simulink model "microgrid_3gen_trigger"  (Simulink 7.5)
settings: Solver=ode23tb  StartTime=0.0  StopTime=20  FixedStep=0.001  RelTol=1e-4
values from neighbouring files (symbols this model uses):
  A = [A_ele, -A_ele, 0    [run_microgrid_3gen_trigger.m]
  B = [2*A_ele,-A_ele,A_ele    [run_microgrid_3gen_trigger.m]
  Ereq1 = 1    [run_microgrid_3gen_trigger.m]
  Ereq2 = 1    [run_microgrid_3gen_trigger.m]
  Ereq3 = 1    [run_microgrid_3gen_trigger.m]
  flag_trigger = 0    [run_microgrid_3gen_trigger.m]
  gen_b = [0.1,1.8,0.5]    [run_microgrid_3gen_trigger.m]
  gen_c = [0.1,0.1,0.1]    [run_microgrid_3gen_trigger.m]
  Ki = 750*160    (= 120000)    [run_microgrid_3gen_trigger.m]
  Kilim = 30    [run_microgrid_3gen_trigger.m]
  Kp = 750*0.001    (= 0.75)    [run_microgrid_3gen_trigger.m]
  Kplim = 0    [run_microgrid_3gen_trigger.m]
  Lgen = 0.00188    [run_microgrid_3gen_trigger.m]
  Lline12 = Lline    (= 1.0345071301e-05)    [run_microgrid_3gen_trigger.m]
  Lline23 = Lline    (= 1.0345071301e-05)    [run_microgrid_3gen_trigger.m]
  Lline31 = Lline    (= 1.0345071301e-05)    [run_microgrid_3gen_trigger.m]
  Lload1 = 0.001/w0    (= 2.65258238486e-06)    [run_microgrid_3gen_trigger.m]
  Lload2 = 0.001/w0    (= 2.65258238486e-06)    [run_microgrid_3gen_trigger.m]
  Lload3 = 0.001/w0    (= 2.65258238486e-06)    [run_microgrid_3gen_trigger.m]
  mP = pi    (= 3.14159265359)    [run_microgrid_3gen_trigger.m]
  mQ = 0.05    [run_microgrid_3gen_trigger.m]
  P_lim_d = [-.4,-.4,-.4]    [run_microgrid_3gen_trigger.m]
  P_lim_u = [.4,.4,.4]    [run_microgrid_3gen_trigger.m]
  Pgen_lim_d = [0.0,0.0,0.0]    [run_microgrid_3gen_trigger.m]
  Pgen_lim_u = [1.0,1.0,1.0]    [run_microgrid_3gen_trigger.m]
  Pmax = 1.0    (= 1)    [run_microgrid_3gen_trigger.m]
  Pmin = 0.0    (= 0)    [run_microgrid_3gen_trigger.m]
  Preq1 = 0.4    [run_microgrid_3gen_trigger.m]    (also in odyssian_4a_plot.m = Preq.signals(1).values; Power_Dispatcher.m = 1)
  Preq2 = 0.8    [run_microgrid_3gen_trigger.m]    (also in odyssian_4a_plot.m = Preq.signals(2).values; Power_Dispatcher.m = 1)
  Preq3 = 0.6    [run_microgrid_3gen_trigger.m]    (also in odyssian_4a_plot.m = Preq.signals(3).values; Power_Dispatcher.m = 1)
  Rline12 = Rline    (= 0)    [run_microgrid_3gen_trigger.m]
  Rline23 = Rline    (= 0)    [run_microgrid_3gen_trigger.m]
  Rline31 = Rline    (= 0)    [run_microgrid_3gen_trigger.m]
  Rload1 = 3    [run_microgrid_3gen_trigger.m]
  Rload2 = 4    [run_microgrid_3gen_trigger.m]
  Rload3 = 6    [run_microgrid_3gen_trigger.m]
  Sbase = 15000    [run_microgrid_3gen_trigger.m]
  t_trigger_start = 3    [run_microgrid_3gen_trigger.m]
  tau_Preq = 0.03    [run_microgrid_3gen_trigger.m]
  tauf = 0.03    [run_microgrid_3gen_trigger.m]
  Vbase = 208/sqrt(3)    [run_microgrid_3gen_trigger.m]
  w0 = 2.0*pi*60    (= 376.991118431)    [run_microgrid_3gen_trigger.m]
  w_d_gen = [w_gen,w_gen,w_gen]    [run_microgrid_3gen_trigger.m]
  w_d_link = [w_line;w_line;w_line]    [run_microgrid_3gen_trigger.m]
  w_u_gen = [w_gen,w_gen,w_gen]    [run_microgrid_3gen_trigger.m]
  w_u_link = [w_line;w_line;w_line]    [run_microgrid_3gen_trigger.m]
libraries: powerlib x73, powerlib_extras x3
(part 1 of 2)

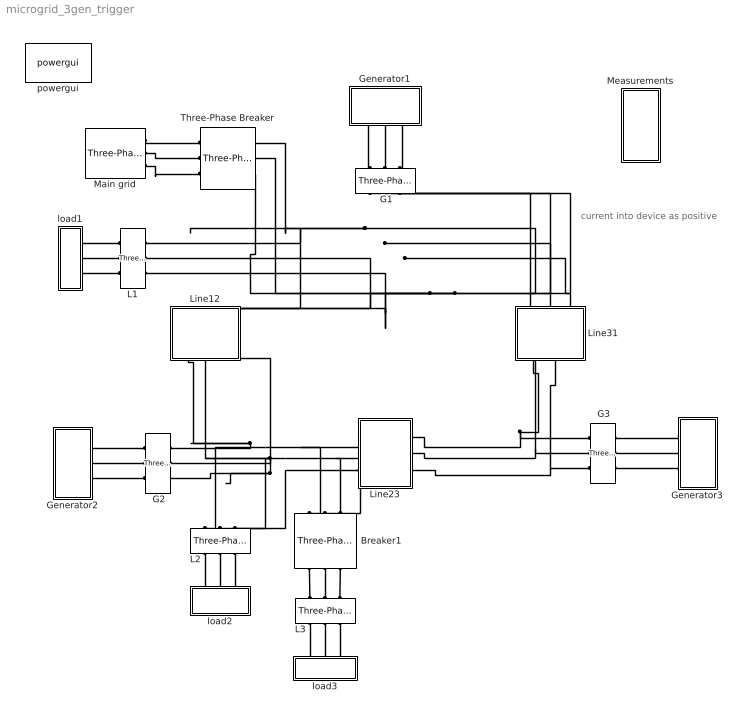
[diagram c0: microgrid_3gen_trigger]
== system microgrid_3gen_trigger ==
  note: current into device as positive
  " G1" : powerlib/Measurements/Three-Phase V-I Measurement  DialogController=POWERSYS.PowerSysDialog  SystemSampleTime=-1  VoltageMeasurement=phase-to-ground  SetLabelV=on  LabelV=v_meas_1  Vpu=off  VpuLL=off  CurrentMeasurement=yes  SetLabelI=on  LabelI=igen_meas_1  Ipu=off  Pbase=100e6  Vbase=500e3  OutputType=Complex  PhasorSimulation=off  PSBequivalent=0
  " G2" : powerlib/Measurements/Three-Phase V-I Measurement  DialogController=POWERSYS.PowerSysDialog  SystemSampleTime=-1  VoltageMeasurement=phase-to-ground  SetLabelV=on  LabelV=v_meas_2  Vpu=off  VpuLL=off  CurrentMeasurement=yes  SetLabelI=on  LabelI=igen_meas_2  Ipu=off  Pbase=100e6  Vbase=500e3  OutputType=Complex  PhasorSimulation=off  PSBequivalent=0
  " G3" : powerlib/Measurements/Three-Phase V-I Measurement  DialogController=POWERSYS.PowerSysDialog  SystemSampleTime=-1  VoltageMeasurement=phase-to-ground  SetLabelV=on  LabelV=v_meas_3  Vpu=off  VpuLL=off  CurrentMeasurement=yes  SetLabelI=on  LabelI=igen_meas_3  Ipu=off  Pbase=100e6  Vbase=500e3  OutputType=Complex  PhasorSimulation=off  PSBequivalent=0
  Breaker1 : powerlib/Elements/Three-Phase Breaker  DialogController=POWERSYS.PowerSysDialog  SystemSampleTime=-1  InitialState=open  SwitchA=on  SwitchB=on  SwitchC=on  SwitchTimes=[10]  External=off  BreakerResistance=0.001  SnubberResistance=1e9  SnubberCapacitance=inf  Measurements=None
  Generator1 : Subsystem
  Generator2 : Subsystem
  Generator3 : Subsystem
  L1 : powerlib/Measurements/Three-Phase V-I Measurement  DialogController=POWERSYS.PowerSysDialog  SystemSampleTime=-1  VoltageMeasurement=phase-to-ground  SetLabelV=on  LabelV=v_meas_load1  Vpu=off  VpuLL=off  CurrentMeasurement=yes  SetLabelI=on  LabelI=iload_meas_1  Ipu=off  Pbase=100e6  Vbase=500e3  OutputType=Complex  PhasorSimulation=off  PSBequivalent=0
  L2 : powerlib/Measurements/Three-Phase V-I Measurement  DialogController=POWERSYS.PowerSysDialog  SystemSampleTime=-1  VoltageMeasurement=phase-to-ground  SetLabelV=on  LabelV=v_meas_load2  Vpu=off  VpuLL=off  CurrentMeasurement=yes  SetLabelI=on  LabelI=iload_meas_2  Ipu=off  Pbase=100e6  Vbase=500e3  OutputType=Complex  PhasorSimulation=off  PSBequivalent=0
  L3 : powerlib/Measurements/Three-Phase V-I Measurement  DialogController=POWERSYS.PowerSysDialog  SystemSampleTime=-1  VoltageMeasurement=phase-to-ground  SetLabelV=on  LabelV=v_meas_load3  Vpu=off  VpuLL=off  CurrentMeasurement=yes  SetLabelI=on  LabelI=iload_meas_3  Ipu=off  Pbase=100e6  Vbase=500e3  OutputType=Complex  PhasorSimulation=off  PSBequivalent=0
  Line12 : Subsystem
  Line23 : Subsystem
  Line31 : Subsystem
  Main grid : powerlib/Electrical Sources/Three-Phase Source  DialogController=POWERSYS.PowerSysDialog  SystemSampleTime=-1  Voltage=208  PhaseAngle=0  Frequency=60  InternalConnection=Yg  SpecifyImpedance=off  Resistance=0.052  Inductance=16.58e-9  ShortCircuitLevel=100e6  BaseVoltage=25e3  XRratio=7
  Measurements : Subsystem
  Three-Phase Breaker : powerlib/Elements/Three-Phase Breaker  DialogController=POWERSYS.PowerSysDialog  SystemSampleTime=-1  InitialState=open  SwitchA=on  SwitchB=on  SwitchC=on  SwitchTimes=[50]  External=off  BreakerResistance=0.001  SnubberResistance=1e9  SnubberCapacitance=inf  Measurements=None
  load1 : Subsystem
  load2 : Subsystem
  load3 : Subsystem
  powergui : powerlib/powergui  Priority=1  SystemSampleTime=-1  SimulationMode=Continuous  SampleTime=50e-6  frequency=60  SPID=off  DisableSnubberDevices=off  DisableRonSwitches=off  DisableVfSwitches=off  SwTol=0  Interpol=off  frequencyindice=0  echomessages=off  HookPort=off  DisplayEquations=off  FunctionMessages=off  EnableUseOfTLC=off  x0status=blocks  RestoreLinks=warning  ResistiveCurrentMeasurement=off  Frange=[0:2:500]  Ylog=off  Xlog=on  ShowGrid=off  save=off  variable=ZData  ZoomFFT=on  StartTime=0.0  cycles=1  DisplayStyle=1  fundamental=60  FreqAxis=off  MaxFrequency=1000  frequencyindicesteady=1  RmsSteady=1  display=off  Ts=0  methode=off
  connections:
  Line23/LConn1 -- Line31/RConn1 -- " G3"/LConn1
  Line23/LConn2 -- Line31/RConn2 -- " G3"/LConn2
  Line23/LConn3 -- Line31/RConn3 -- " G3"/LConn3
  Line23/RConn1 -- " G2"/LConn1 -- Line12/LConn1 -- L2/LConn1 -- Breaker1/LConn1
  Line23/RConn2 -- " G2"/LConn2 -- Line12/LConn2 -- L2/LConn2 -- Breaker1/LConn2
  Line23/RConn3 -- L2/LConn3 -- " G2"/LConn3 -- Line12/LConn3 -- Breaker1/LConn3
  Generator3/RConn3 -- " G3"/RConn3
  Generator3/RConn2 -- " G3"/RConn2
  Generator3/RConn1 -- " G3"/RConn1
  Line31/LConn1 -- " G1"/LConn1 -- L1/LConn1 -- Line12/RConn1 -- Three-Phase Breaker/RConn1
  Line31/LConn2 -- " G1"/LConn2 -- L1/LConn2 -- Line12/RConn2 -- Three-Phase Breaker/RConn2
  Line31/LConn3 -- " G1"/LConn3 -- L1/LConn3 -- Line12/RConn3 -- Three-Phase Breaker/RConn3
  load1/LConn1 -- L1/RConn1
  load1/LConn2 -- L1/RConn2
  load1/LConn3 -- L1/RConn3
  L2/RConn3 -- load2/LConn3
  L2/RConn2 -- load2/LConn2
  L2/RConn1 -- load2/LConn1
  Main grid/RConn1 -- Three-Phase Breaker/LConn1
  Main grid/RConn2 -- Three-Phase Breaker/LConn2
  Main grid/RConn3 -- Three-Phase Breaker/LConn3
  Generator2/RConn2 -- " G2"/RConn2
  Generator2/RConn3 -- " G2"/RConn3
  Generator2/RConn1 -- " G2"/RConn1
  Breaker1/RConn3 -- L3/LConn3
  Breaker1/RConn2 -- L3/LConn2
  Breaker1/RConn1 -- L3/LConn1
  L3/RConn1 -- load3/LConn1
  L3/RConn2 -- load3/LConn2
  L3/RConn3 -- load3/LConn3
  Generator1/RConn2 -- " G1"/RConn2
  Generator1/RConn3 -- " G1"/RConn3
  Generator1/RConn1 -- " G1"/RConn1

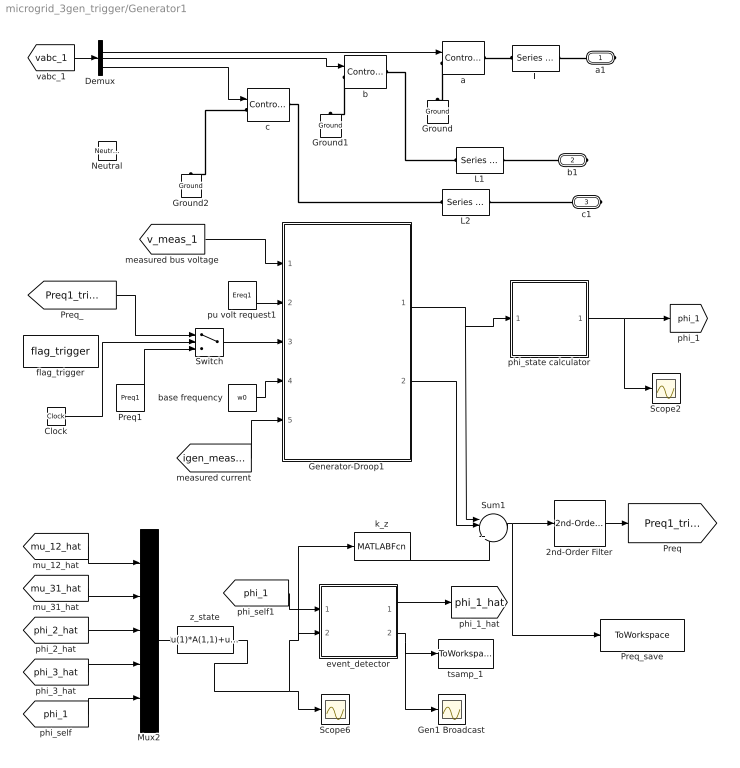
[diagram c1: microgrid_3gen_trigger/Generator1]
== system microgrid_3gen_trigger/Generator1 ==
  2nd-Order Filter : powerlib_extras/Control  Blocks/2nd-Order Filter  DialogController=POWERSYS.PowerSysDialog  SystemSampleTime=-1  FilterType=Lowpass  Fo=20  Zeta=0.707  Initialize=off  Vac_Init=[1 45 60]  Vdc_Init=-0.5  PlotResponse=off  param1=[1 150 1]
  Clock : Clock
  Demux : Demux  Outputs=3
  Gen1 Broadcast : Scope
  Generator-Droop1 : Subsystem
  Ground : powerlib/Elements/Ground  DialogController=POWERSYS.PowerSysDialog  PhysicalDomain=powersysdomain  SubClassName=unknown  LeftPortType=p1  RightPortType=p1  LConnTagsString=a
  Ground1 : powerlib/Elements/Ground  DialogController=POWERSYS.PowerSysDialog  PhysicalDomain=powersysdomain  SubClassName=unknown  LeftPortType=p1  RightPortType=p1  LConnTagsString=a
  Ground2 : powerlib/Elements/Ground  DialogController=POWERSYS.PowerSysDialog  PhysicalDomain=powersysdomain  SubClassName=unknown  LeftPortType=p1  RightPortType=p1  LConnTagsString=a
  L : powerlib/Elements/Series RLC Branch  DialogController=POWERSYS.PowerSysDialog  PhysicalDomain=powersysdomain  SubClassName=unknown  LeftPortType=p1  RightPortType=p1  LConnTagsString=__new0  RConnTagsString=__new0  BranchType=L  Resistance=1  Inductance=Lgen  SetiL0=off  InitialCurrent=0  Capacitance=1e-6  Setx0=off  InitialVoltage=0  Measurements=None
  L1 : powerlib/Elements/Series RLC Branch  DialogController=POWERSYS.PowerSysDialog  PhysicalDomain=powersysdomain  SubClassName=unknown  LeftPortType=p1  RightPortType=p1  LConnTagsString=__new0  RConnTagsString=__new0  BranchType=L  Resistance=1  Inductance=Lgen  SetiL0=off  InitialCurrent=0  Capacitance=1e-6  Setx0=off  InitialVoltage=0  Measurements=None
  L2 : powerlib/Elements/Series RLC Branch  DialogController=POWERSYS.PowerSysDialog  PhysicalDomain=powersysdomain  SubClassName=unknown  LeftPortType=p1  RightPortType=p1  LConnTagsString=__new0  RConnTagsString=__new0  BranchType=L  Resistance=1  Inductance=Lgen  SetiL0=off  InitialCurrent=0  Capacitance=1e-6  Setx0=off  InitialVoltage=0  Measurements=None
  Mux2 : Mux  Inputs=5
  Neutral : powerlib/Elements/Neutral  DialogController=POWERSYS.PowerSysDialog  PhysicalDomain=powersysdomain  SubClassName=unknown  LeftPortType=p1  RightPortType=p1  LConnTagsString=a  NodeNumber=10
  Preq1 : Constant  Value=Preq1  OutDataType=sfix(16)  OutScaling=2^0
  Preq_save : ToWorkspace  VariableName=Preq1_trigger  SampleTime=-1  SaveFormat=Array
  Scope2 : Scope
  Scope6 : Scope
  Sum1 : Sum  Inputs=|++++  OutDataType=sfix(16)  OutScaling=2^0
  Switch : Switch  Criteria=u2 > Threshold  Threshold=t_trigger_start  OutDataType=fixdt(1, 16)  OutScaling=2^0
  a : powerlib/Electrical Sources/Controlled Voltage Source  DialogController=POWERSYS.PowerSysDialog  SystemSampleTime=-1  Initialize=on  Source_Type=AC  Amplitude=0  Phase=0  Frequency=0  Measurements=None
  b : powerlib/Electrical Sources/Controlled Voltage Source  DialogController=POWERSYS.PowerSysDialog  SystemSampleTime=-1  Initialize=on  Source_Type=AC  Amplitude=0  Phase=0  Frequency=0  Measurements=None
  base frequency : Constant  Value=w0  OutDataType=sfix(16)  OutScaling=2^0
  c : powerlib/Electrical Sources/Controlled Voltage Source  DialogController=POWERSYS.PowerSysDialog  SystemSampleTime=-1  Initialize=on  Source_Type=AC  Amplitude=0  Phase=0  Frequency=0  Measurements=None
  event_detector : Subsystem
  flag_trigger : Constant  Value=flag_trigger  OutDataType=sfix(16)  OutScaling=2^0
  k_z : MATLABFcn  MATLABFcn=k_z
  phi_state calculator : Subsystem
  pu volt request1 : Constant  Value=Ereq1  OutDataType=sfix(16)  OutScaling=2^0
  tsamp_1 : ToWorkspace  VariableName=tsamp_1  SampleTime=-1  SaveFormat=Array
  z_state : Fcn  Expr=u(1)*A(1,1)+u(2)*A(3,1)+u(3)*B(2,1)+u(4)*B(3,1)+u(5)*B(1,1)
  a1 : PMIOPort  Port=1  Side=Right
  b1 : PMIOPort  Port=2  Side=Right
  c1 : PMIOPort  Port=3  Side=Right
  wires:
  Demux/1 -> a/1
  Demux/2 -> b/1
  Demux/3 -> c/1
  [vabc_1] -> Demux/1
  pu volt request1/1 -> Generator-Droop1/2(E_req)
  base frequency/1 -> Generator-Droop1/4(w0)
  [v_meas_1] -> Generator-Droop1/1(v_bus_meas)
  [igen_meas_1] -> Generator-Droop1/5(i_meas)
  Generator-Droop1/1(Pmeas) -> Sum1/1, phi_state calculator/1(P_meas)
  [phi_1] -> event_detector/1(phi)
  event_detector/1(phi_hat) -> [phi_1_hat]
  event_detector/2(tsamp) -> tsamp_1/1, Gen1 Broadcast/1
  Sum1/1 -> Preq_save/1, 2nd-Order Filter/1
  Switch/1 -> Generator-Droop1/3(P_req)
  Preq1/1 -> Switch/3
  [Preq1_trigger] -> Switch/1
  Clock/1 -> Switch/2
  phi_state calculator/1(phi) -> [phi_1], Scope2/1
  z_state/1 -> Scope6/1, event_detector/2(z), k_z/1
  k_z/1 -> Sum1/4
  ? -> Sum1/3
  Generator-Droop1/2(Pmm) -> Sum1/2
  2nd-Order Filter/1 -> [Preq1_trigger]
  [mu_12_hat] -> Mux2/1
  [mu_31_hat] -> Mux2/2
  [phi_2_hat] -> Mux2/3
  [phi_3_hat] -> Mux2/4
  [phi_1] -> Mux2/5
  Mux2/1 -> z_state/1
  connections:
  L/RConn1 -- a1/RConn1
  L/LConn1 -- a/RConn1
  L1/RConn1 -- b1/RConn1
  b/RConn1 -- L1/LConn1
  L2/RConn1 -- c1/RConn1
  c/RConn1 -- L2/LConn1
  c/LConn1 -- Ground2/LConn1
  b/LConn1 -- Ground1/LConn1
  a/LConn1 -- Ground/LConn1

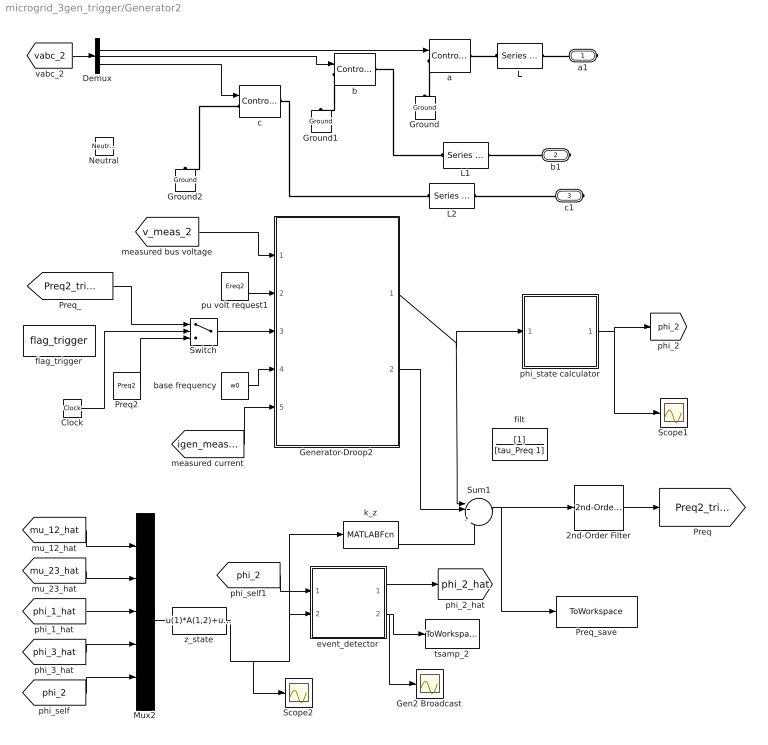
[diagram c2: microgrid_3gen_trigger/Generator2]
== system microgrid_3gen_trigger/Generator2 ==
  2nd-Order Filter : powerlib_extras/Control  Blocks/2nd-Order Filter  DialogController=POWERSYS.PowerSysDialog  SystemSampleTime=-1  FilterType=Lowpass  Fo=20  Zeta=0.707  Initialize=off  Vac_Init=[1 45 60]  Vdc_Init=-0.5  PlotResponse=off  param1=[1 150 1]
  Clock : Clock
  Demux : Demux  Outputs=3
  Gen2 Broadcast : Scope
  Generator-Droop2 : Subsystem
  Ground : powerlib/Elements/Ground  DialogController=POWERSYS.PowerSysDialog  PhysicalDomain=powersysdomain  SubClassName=unknown  LeftPortType=p1  RightPortType=p1  LConnTagsString=a
  Ground1 : powerlib/Elements/Ground  DialogController=POWERSYS.PowerSysDialog  PhysicalDomain=powersysdomain  SubClassName=unknown  LeftPortType=p1  RightPortType=p1  LConnTagsString=a
  Ground2 : powerlib/Elements/Ground  DialogController=POWERSYS.PowerSysDialog  PhysicalDomain=powersysdomain  SubClassName=unknown  LeftPortType=p1  RightPortType=p1  LConnTagsString=a
  L : powerlib/Elements/Series RLC Branch  DialogController=POWERSYS.PowerSysDialog  PhysicalDomain=powersysdomain  SubClassName=unknown  LeftPortType=p1  RightPortType=p1  LConnTagsString=__new0  RConnTagsString=__new0  BranchType=L  Resistance=1  Inductance=Lgen  SetiL0=off  InitialCurrent=0  Capacitance=1e-6  Setx0=off  InitialVoltage=0  Measurements=None
  L1 : powerlib/Elements/Series RLC Branch  DialogController=POWERSYS.PowerSysDialog  PhysicalDomain=powersysdomain  SubClassName=unknown  LeftPortType=p1  RightPortType=p1  LConnTagsString=__new0  RConnTagsString=__new0  BranchType=L  Resistance=1  Inductance=Lgen  SetiL0=off  InitialCurrent=0  Capacitance=1e-6  Setx0=off  InitialVoltage=0  Measurements=None
  L2 : powerlib/Elements/Series RLC Branch  DialogController=POWERSYS.PowerSysDialog  PhysicalDomain=powersysdomain  SubClassName=unknown  LeftPortType=p1  RightPortType=p1  LConnTagsString=__new0  RConnTagsString=__new0  BranchType=L  Resistance=1  Inductance=Lgen  SetiL0=off  InitialCurrent=0  Capacitance=1e-6  Setx0=off  InitialVoltage=0  Measurements=None
  Mux2 : Mux  Inputs=5
  Neutral : powerlib/Elements/Neutral  DialogController=POWERSYS.PowerSysDialog  PhysicalDomain=powersysdomain  SubClassName=unknown  LeftPortType=p1  RightPortType=p1  LConnTagsString=a  NodeNumber=10
  Preq2 : Constant  Value=Preq2  OutDataType=sfix(16)  OutScaling=2^0
  Preq_save : ToWorkspace  VariableName=Preq2_trigger  SampleTime=-1  SaveFormat=Array
  Scope1 : Scope
  Scope2 : Scope
  Sum1 : Sum  Inputs=|++++  OutDataType=sfix(16)  OutScaling=2^0
  Switch : Switch  Criteria=u2 > Threshold  Threshold=t_trigger_start  OutDataType=fixdt(1, 16)  OutScaling=2^0
  a : powerlib/Electrical Sources/Controlled Voltage Source  DialogController=POWERSYS.PowerSysDialog  SystemSampleTime=-1  Initialize=on  Source_Type=AC  Amplitude=0  Phase=0  Frequency=0  Measurements=None
  b : powerlib/Electrical Sources/Controlled Voltage Source  DialogController=POWERSYS.PowerSysDialog  SystemSampleTime=-1  Initialize=on  Source_Type=AC  Amplitude=0  Phase=0  Frequency=0  Measurements=None
  base frequency : Constant  Value=w0  OutDataType=sfix(16)  OutScaling=2^0
  c : powerlib/Electrical Sources/Controlled Voltage Source  DialogController=POWERSYS.PowerSysDialog  SystemSampleTime=-1  Initialize=on  Source_Type=AC  Amplitude=0  Phase=0  Frequency=0  Measurements=None
  event_detector : Subsystem
  filt : TransferFcn  Denominator=[tau_Preq 1]
  flag_trigger : Constant  Value=flag_trigger  OutDataType=sfix(16)  OutScaling=2^0
  k_z : MATLABFcn  MATLABFcn=k_z
  phi_state calculator : Subsystem
  pu volt request1 : Constant  Value=Ereq2  OutDataType=sfix(16)  OutScaling=2^0
  tsamp_2 : ToWorkspace  VariableName=tsamp_2  SampleTime=-1  SaveFormat=Array
  z_state : Fcn  Expr=u(1)*A(1,2)+u(2)*A(2,2)+u(3)*B(1,2)+u(4)*B(3,2)+u(5)*B(2,2)
  a1 : PMIOPort  Port=1  Side=Right
  b1 : PMIOPort  Port=2  Side=Right
  c1 : PMIOPort  Port=3  Side=Right
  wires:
  Demux/1 -> a/1
  Demux/2 -> b/1
  Demux/3 -> c/1
  [vabc_2] -> Demux/1
  pu volt request1/1 -> Generator-Droop2/2(E_req)
  base frequency/1 -> Generator-Droop2/4(w0)
  [v_meas_2] -> Generator-Droop2/1(v_bus_meas)
  [igen_meas_2] -> Generator-Droop2/5(i_meas)
  Generator-Droop2/1(Pmeas) -> Sum1/1, phi_state calculator/1(P_meas)
  [phi_2] -> event_detector/1(phi)
  event_detector/1(phi_hat) -> [phi_2_hat]
  event_detector/2(tsamp) -> tsamp_2/1, Gen2 Broadcast/1
  Sum1/1 -> Preq_save/1, 2nd-Order Filter/1
  Switch/1 -> Generator-Droop2/3(P_req)
  Preq2/1 -> Switch/3
  [Preq2_trigger] -> Switch/1
  Clock/1 -> Switch/2
  phi_state calculator/1(phi) -> [phi_2], Scope1/1
  z_state/1 -> event_detector/2(z), k_z/1, Scope2/1
  k_z/1 -> Sum1/4
  ? -> Sum1/3
  Generator-Droop2/2(Pmm) -> Sum1/2
  2nd-Order Filter/1 -> [Preq2_trigger]
  [mu_12_hat] -> Mux2/1
  [mu_23_hat] -> Mux2/2
  [phi_1_hat] -> Mux2/3
  [phi_3_hat] -> Mux2/4
  [phi_2] -> Mux2/5
  Mux2/1 -> z_state/1
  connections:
  L/RConn1 -- a1/RConn1
  L/LConn1 -- a/RConn1
  L1/RConn1 -- b1/RConn1
  b/RConn1 -- L1/LConn1
  L2/RConn1 -- c1/RConn1
  c/RConn1 -- L2/LConn1
  c/LConn1 -- Ground2/LConn1
  b/LConn1 -- Ground1/LConn1
  a/LConn1 -- Ground/LConn1

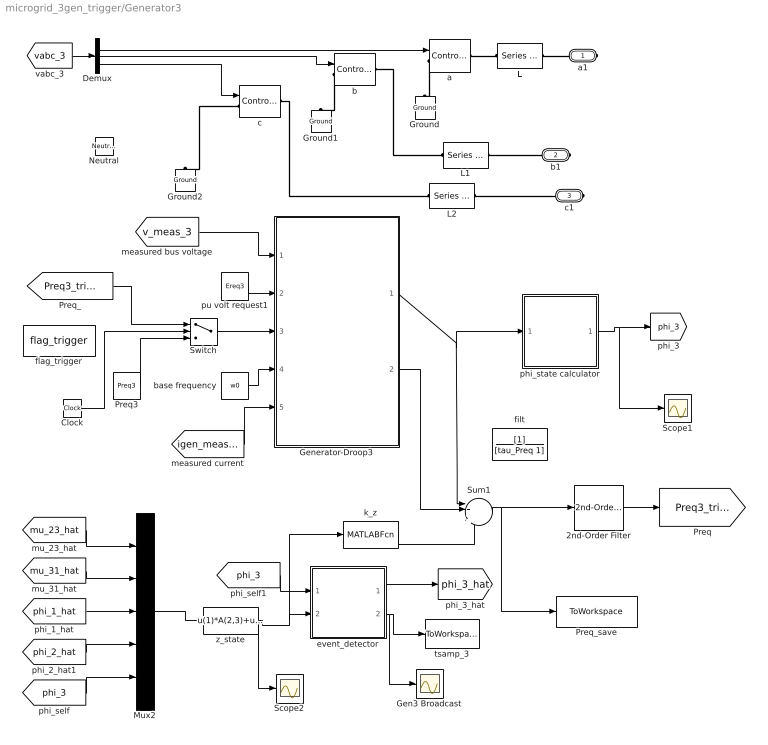
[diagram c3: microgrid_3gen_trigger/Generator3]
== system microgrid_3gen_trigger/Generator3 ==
  2nd-Order Filter : powerlib_extras/Control  Blocks/2nd-Order Filter  DialogController=POWERSYS.PowerSysDialog  SystemSampleTime=-1  FilterType=Lowpass  Fo=20  Zeta=0.707  Initialize=off  Vac_Init=[1 45 60]  Vdc_Init=-0.5  PlotResponse=off  param1=[1 150 1]
  Clock : Clock
  Demux : Demux  Outputs=3
  Gen3 Broadcast : Scope
  Generator-Droop3 : Subsystem
  Ground : powerlib/Elements/Ground  DialogController=POWERSYS.PowerSysDialog  PhysicalDomain=powersysdomain  SubClassName=unknown  LeftPortType=p1  RightPortType=p1  LConnTagsString=a
  Ground1 : powerlib/Elements/Ground  DialogController=POWERSYS.PowerSysDialog  PhysicalDomain=powersysdomain  SubClassName=unknown  LeftPortType=p1  RightPortType=p1  LConnTagsString=a
  Ground2 : powerlib/Elements/Ground  DialogController=POWERSYS.PowerSysDialog  PhysicalDomain=powersysdomain  SubClassName=unknown  LeftPortType=p1  RightPortType=p1  LConnTagsString=a
  L : powerlib/Elements/Series RLC Branch  DialogController=POWERSYS.PowerSysDialog  PhysicalDomain=powersysdomain  SubClassName=unknown  LeftPortType=p1  RightPortType=p1  LConnTagsString=__new0  RConnTagsString=__new0  BranchType=L  Resistance=1  Inductance=Lgen  SetiL0=off  InitialCurrent=0  Capacitance=1e-6  Setx0=off  InitialVoltage=0  Measurements=None
  L1 : powerlib/Elements/Series RLC Branch  DialogController=POWERSYS.PowerSysDialog  PhysicalDomain=powersysdomain  SubClassName=unknown  LeftPortType=p1  RightPortType=p1  LConnTagsString=__new0  RConnTagsString=__new0  BranchType=L  Resistance=1  Inductance=Lgen  SetiL0=off  InitialCurrent=0  Capacitance=1e-6  Setx0=off  InitialVoltage=0  Measurements=None
  L2 : powerlib/Elements/Series RLC Branch  DialogController=POWERSYS.PowerSysDialog  PhysicalDomain=powersysdomain  SubClassName=unknown  LeftPortType=p1  RightPortType=p1  LConnTagsString=__new0  RConnTagsString=__new0  BranchType=L  Resistance=1  Inductance=Lgen  SetiL0=off  InitialCurrent=0  Capacitance=1e-6  Setx0=off  InitialVoltage=0  Measurements=None
  Mux2 : Mux  Inputs=5
  Neutral : powerlib/Elements/Neutral  DialogController=POWERSYS.PowerSysDialog  PhysicalDomain=powersysdomain  SubClassName=unknown  LeftPortType=p1  RightPortType=p1  LConnTagsString=a  NodeNumber=10
  Preq3 : Constant  Value=Preq3  OutDataType=sfix(16)  OutScaling=2^0
  Preq_save : ToWorkspace  VariableName=Preq3_trigger  SampleTime=-1  SaveFormat=Array
  Scope1 : Scope
  Scope2 : Scope
  Sum1 : Sum  Inputs=|++++  OutDataType=sfix(16)  OutScaling=2^0
  Switch : Switch  Criteria=u2 > Threshold  Threshold=t_trigger_start  OutDataType=fixdt(1, 16)  OutScaling=2^0
  a : powerlib/Electrical Sources/Controlled Voltage Source  DialogController=POWERSYS.PowerSysDialog  SystemSampleTime=-1  Initialize=on  Source_Type=AC  Amplitude=0  Phase=0  Frequency=0  Measurements=None
  b : powerlib/Electrical Sources/Controlled Voltage Source  DialogController=POWERSYS.PowerSysDialog  SystemSampleTime=-1  Initialize=on  Source_Type=AC  Amplitude=0  Phase=0  Frequency=0  Measurements=None
  base frequency : Constant  Value=w0  OutDataType=sfix(16)  OutScaling=2^0
  c : powerlib/Electrical Sources/Controlled Voltage Source  DialogController=POWERSYS.PowerSysDialog  SystemSampleTime=-1  Initialize=on  Source_Type=AC  Amplitude=0  Phase=0  Frequency=0  Measurements=None
  event_detector : Subsystem
  filt : TransferFcn  Denominator=[tau_Preq 1]
  flag_trigger : Constant  Value=flag_trigger  OutDataType=sfix(16)  OutScaling=2^0
  k_z : MATLABFcn  MATLABFcn=k_z
  phi_state calculator : Subsystem
  pu volt request1 : Constant  Value=Ereq3  OutDataType=sfix(16)  OutScaling=2^0
  tsamp_3 : ToWorkspace  VariableName=tsamp_3  SampleTime=-1  SaveFormat=Array
  z_state : Fcn  Expr=u(1)*A(2,3)+u(2)*A(3,3)+u(3)*B(1,3)+u(4)*B(2,3)+u(5)*B(3,3)
  a1 : PMIOPort  Port=1  Side=Right
  b1 : PMIOPort  Port=2  Side=Right
  c1 : PMIOPort  Port=3  Side=Right
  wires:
  Demux/1 -> a/1
  Demux/2 -> b/1
  Demux/3 -> c/1
  [vabc_3] -> Demux/1
  pu volt request1/1 -> Generator-Droop3/2(E_req)
  base frequency/1 -> Generator-Droop3/4(w0)
  [v_meas_3] -> Generator-Droop3/1(v_bus_meas)
  [igen_meas_3] -> Generator-Droop3/5(i_meas)
  Generator-Droop3/1(Pmeas) -> Sum1/1, phi_state calculator/1(P_meas)
  [phi_3] -> event_detector/1(phi)
  event_detector/1(phi_hat) -> [phi_3_hat]
  event_detector/2(tsamp) -> tsamp_3/1, Gen3 Broadcast/1
  Sum1/1 -> Preq_save/1, 2nd-Order Filter/1
  Switch/1 -> Generator-Droop3/3(P_req)
  Preq3/1 -> Switch/3
  [Preq3_trigger] -> Switch/1
  Clock/1 -> Switch/2
  phi_state calculator/1(phi) -> [phi_3], Scope1/1
  z_state/1 -> event_detector/2(z), k_z/1, Scope2/1
  k_z/1 -> Sum1/4
  ? -> Sum1/3
  Generator-Droop3/2(Pmm) -> Sum1/2
  2nd-Order Filter/1 -> [Preq3_trigger]
  [mu_23_hat] -> Mux2/1
  [mu_31_hat] -> Mux2/2
  [phi_1_hat] -> Mux2/3
  [phi_2_hat] -> Mux2/4
  [phi_3] -> Mux2/5
  Mux2/1 -> z_state/1
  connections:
  L/RConn1 -- a1/RConn1
  L/LConn1 -- a/RConn1
  L1/RConn1 -- b1/RConn1
  b/RConn1 -- L1/LConn1
  L2/RConn1 -- c1/RConn1
  c/RConn1 -- L2/LConn1
  c/LConn1 -- Ground2/LConn1
  b/LConn1 -- Ground1/LConn1
  a/LConn1 -- Ground/LConn1

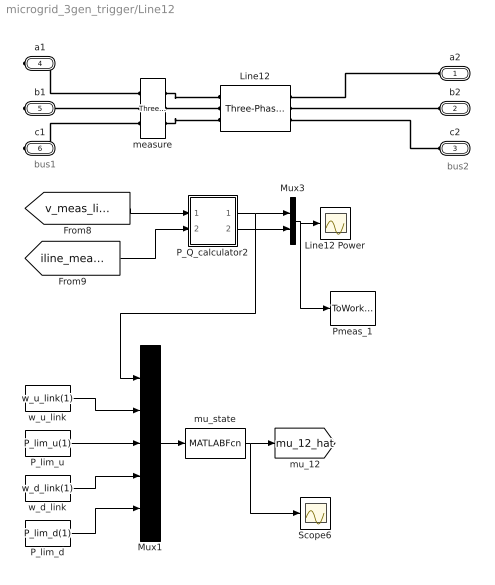
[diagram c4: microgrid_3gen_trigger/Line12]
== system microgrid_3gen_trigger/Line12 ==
  note: bus1
  note: bus2
  Line12 : powerlib/Elements/Three-Phase Series RLC Branch  DialogController=POWERSYS.PowerSysDialog  PhysicalDomain=powersysdomain  SubClassName=unknown  LeftPortType=p1  RightPortType=p1  LConnTagsString=A|B|C  RConnTagsString=A|B|C  BranchType=RL  Resistance=Rline12  Inductance=Lline12  Capacitance=1e-6  Measurements=None
  Line12 Power : Scope
  Mux1 : Mux  Inputs=5
  Mux3 : Mux  Inputs=2
  P_Q_calculator2 : Subsystem
  P_lim_d : Constant  Value=P_lim_d(1)  OutDataType=sfix(16)  OutScaling=2^0
  P_lim_u : Constant  Value=P_lim_u(1)  OutDataType=sfix(16)  OutScaling=2^0
  Pmeas_1 : ToWorkspace  VariableName=PQline_12  SampleTime=-1  SaveFormat=Array
  Scope6 : Scope
  measure : powerlib/Measurements/Three-Phase V-I Measurement  DialogController=POWERSYS.PowerSysDialog  SystemSampleTime=-1  VoltageMeasurement=phase-to-ground  SetLabelV=on  LabelV=v_meas_line12  Vpu=off  VpuLL=off  CurrentMeasurement=yes  SetLabelI=on  LabelI=iline_meas_12  Ipu=off  Pbase=100e6  Vbase=500e3  OutputType=Complex  PhasorSimulation=off  PSBequivalent=0
  mu_state : MATLABFcn  MATLABFcn=mu_state
  w_d_link : Constant  Value=w_d_link(1)  OutDataType=sfix(16)  OutScaling=2^0
  w_u_link : Constant  Value=w_u_link(1)  OutDataType=sfix(16)  OutScaling=2^0
  a2 : PMIOPort  Port=1  Side=Left
  b2 : PMIOPort  Port=2  Side=Left
  c2 : PMIOPort  Port=3  Side=Left
  a1 : PMIOPort  Port=4  Side=Right
  b1 : PMIOPort  Port=5  Side=Right
  c1 : PMIOPort  Port=6  Side=Right
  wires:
  [v_meas_line12] -> P_Q_calculator2/1(v)
  [iline_meas_12] -> P_Q_calculator2/2(i)
  Mux3/1 -> Line12 Power/1, Pmeas_1/1
  P_Q_calculator2/1(P) -> Mux3/1, Mux1/1
  P_Q_calculator2/2(Q) -> Mux3/2
  Mux1/1 -> mu_state/1
  w_u_link/1 -> Mux1/2
  P_lim_u/1 -> Mux1/3
  w_d_link/1 -> Mux1/4
  P_lim_d/1 -> Mux1/5
  mu_state/1 -> [mu_12_hat], Scope6/1
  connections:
  Line12/LConn1 -- a2/RConn1
  Line12/LConn2 -- b2/RConn1
  Line12/LConn3 -- c2/RConn1
  measure/RConn1 -- Line12/RConn1
  measure/RConn2 -- Line12/RConn2
  measure/RConn3 -- Line12/RConn3
  a1/RConn1 -- measure/LConn1
  b1/RConn1 -- measure/LConn2
  c1/RConn1 -- measure/LConn3

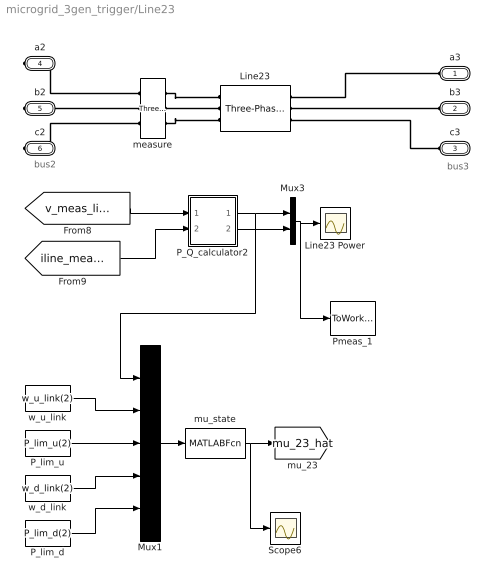
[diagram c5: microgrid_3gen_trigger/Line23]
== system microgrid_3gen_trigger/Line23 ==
  note: bus2
  note: bus3
  Line23 : powerlib/Elements/Three-Phase Series RLC Branch  DialogController=POWERSYS.PowerSysDialog  PhysicalDomain=powersysdomain  SubClassName=unknown  LeftPortType=p1  RightPortType=p1  LConnTagsString=A|B|C  RConnTagsString=A|B|C  BranchType=RL  Resistance=Rline23  Inductance=Lline23  Capacitance=1e-6  Measurements=None
  Line23 Power : Scope
  Mux1 : Mux  Inputs=5
  Mux3 : Mux  Inputs=2
  P_Q_calculator2 : Subsystem
  P_lim_d : Constant  Value=P_lim_d(2)  OutDataType=sfix(16)  OutScaling=2^0
  P_lim_u : Constant  Value=P_lim_u(2)  OutDataType=sfix(16)  OutScaling=2^0
  Pmeas_1 : ToWorkspace  VariableName=PQline_23  SampleTime=-1  SaveFormat=Array
  Scope6 : Scope
  measure : powerlib/Measurements/Three-Phase V-I Measurement  DialogController=POWERSYS.PowerSysDialog  SystemSampleTime=-1  VoltageMeasurement=phase-to-ground  SetLabelV=on  LabelV=v_meas_line23  Vpu=off  VpuLL=off  CurrentMeasurement=yes  SetLabelI=on  LabelI=iline_meas_23  Ipu=off  Pbase=100e6  Vbase=500e3  OutputType=Complex  PhasorSimulation=off  PSBequivalent=0
  mu_state : MATLABFcn  MATLABFcn=mu_state
  w_d_link : Constant  Value=w_d_link(2)  OutDataType=sfix(16)  OutScaling=2^0
  w_u_link : Constant  Value=w_u_link(2)  OutDataType=sfix(16)  OutScaling=2^0
  a3 : PMIOPort  Port=1  Side=Left
  b3 : PMIOPort  Port=2  Side=Left
  c3 : PMIOPort  Port=3  Side=Left
  a2 : PMIOPort  Port=4  Side=Right
  b2 : PMIOPort  Port=5  Side=Right
  c2 : PMIOPort  Port=6  Side=Right
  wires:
  [v_meas_line23] -> P_Q_calculator2/1(v)
  [iline_meas_23] -> P_Q_calculator2/2(i)
  Mux3/1 -> Line23 Power/1, Pmeas_1/1
  P_Q_calculator2/1(P) -> Mux3/1, Mux1/1
  P_Q_calculator2/2(Q) -> Mux3/2
  Mux1/1 -> mu_state/1
  w_u_link/1 -> Mux1/2
  P_lim_u/1 -> Mux1/3
  w_d_link/1 -> Mux1/4
  P_lim_d/1 -> Mux1/5
  mu_state/1 -> [mu_23_hat], Scope6/1
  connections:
  Line23/LConn1 -- a3/RConn1
  Line23/LConn2 -- b3/RConn1
  Line23/LConn3 -- c3/RConn1
  measure/RConn1 -- Line23/RConn1
  measure/RConn2 -- Line23/RConn2
  measure/RConn3 -- Line23/RConn3
  a2/RConn1 -- measure/LConn1
  b2/RConn1 -- measure/LConn2
  c2/RConn1 -- measure/LConn3

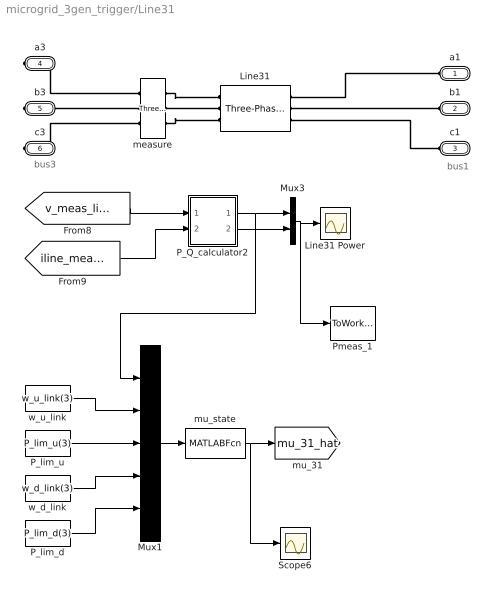
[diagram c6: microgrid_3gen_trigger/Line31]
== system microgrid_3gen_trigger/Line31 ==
  note: bus3
  note: bus1
  Line31 : powerlib/Elements/Three-Phase Series RLC Branch  DialogController=POWERSYS.PowerSysDialog  PhysicalDomain=powersysdomain  SubClassName=unknown  LeftPortType=p1  RightPortType=p1  LConnTagsString=A|B|C  RConnTagsString=A|B|C  BranchType=RL  Resistance=Rline31  Inductance=Lline31  Capacitance=1e-6  Measurements=None
  Line31 Power : Scope
  Mux1 : Mux  Inputs=5
  Mux3 : Mux  Inputs=2
  P_Q_calculator2 : Subsystem
  P_lim_d : Constant  Value=P_lim_d(3)  OutDataType=sfix(16)  OutScaling=2^0
  P_lim_u : Constant  Value=P_lim_u(3)  OutDataType=sfix(16)  OutScaling=2^0
  Pmeas_1 : ToWorkspace  VariableName=PQline_31  SampleTime=-1  SaveFormat=Array
  Scope6 : Scope
  measure : powerlib/Measurements/Three-Phase V-I Measurement  DialogController=POWERSYS.PowerSysDialog  SystemSampleTime=-1  VoltageMeasurement=phase-to-ground  SetLabelV=on  LabelV=v_meas_line31  Vpu=off  VpuLL=off  CurrentMeasurement=yes  SetLabelI=on  LabelI=iline_meas_31  Ipu=off  Pbase=100e6  Vbase=500e3  OutputType=Complex  PhasorSimulation=off  PSBequivalent=0
  mu_state : MATLABFcn  MATLABFcn=mu_state
  w_d_link : Constant  Value=w_d_link(3)  OutDataType=sfix(16)  OutScaling=2^0
  w_u_link : Constant  Value=w_u_link(3)  OutDataType=sfix(16)  OutScaling=2^0
  a1 : PMIOPort  Port=1  Side=Left
  b1 : PMIOPort  Port=2  Side=Left
  c1 : PMIOPort  Port=3  Side=Left
  a3 : PMIOPort  Port=4  Side=Right
  b3 : PMIOPort  Port=5  Side=Right
  c3 : PMIOPort  Port=6  Side=Right
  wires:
  [v_meas_line31] -> P_Q_calculator2/1(v)
  [iline_meas_31] -> P_Q_calculator2/2(i)
  Mux3/1 -> Line31 Power/1, Pmeas_1/1
  P_Q_calculator2/1(P) -> Mux3/1, Mux1/1
  P_Q_calculator2/2(Q) -> Mux3/2
  Mux1/1 -> mu_state/1
  w_u_link/1 -> Mux1/2
  P_lim_u/1 -> Mux1/3
  w_d_link/1 -> Mux1/4
  P_lim_d/1 -> Mux1/5
  mu_state/1 -> [mu_31_hat], Scope6/1
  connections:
  Line31/LConn1 -- a1/RConn1
  Line31/LConn2 -- b1/RConn1
  Line31/LConn3 -- c1/RConn1
  measure/RConn1 -- Line31/RConn1
  measure/RConn2 -- Line31/RConn2
  measure/RConn3 -- Line31/RConn3
  a3/RConn1 -- measure/LConn1
  b3/RConn1 -- measure/LConn2
  c3/RConn1 -- measure/LConn3

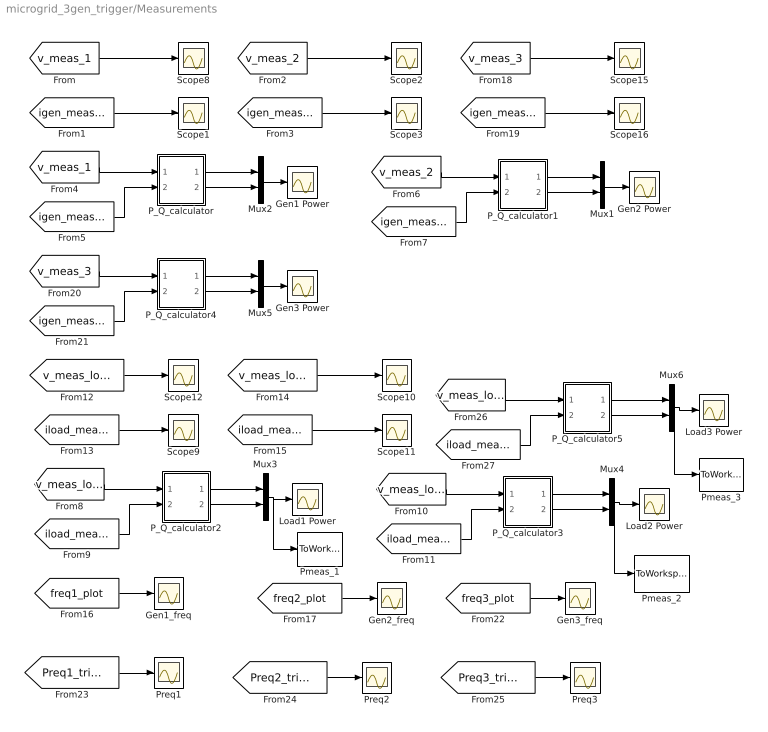
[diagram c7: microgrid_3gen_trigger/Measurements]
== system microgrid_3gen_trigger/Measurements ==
  Gen1 Power : Scope
  Gen1_freq : Scope
  Gen2 Power : Scope
  Gen2_freq : Scope
  Gen3 Power : Scope
  Gen3_freq : Scope
  Load1 Power : Scope
  Load2 Power : Scope
  Load3 Power : Scope
  Mux{1..6} (6 alike) : Mux  Inputs=2
  P_Q_calculator : Subsystem
  P_Q_calculator1 : Subsystem
  P_Q_calculator2 : Subsystem
  P_Q_calculator3 : Subsystem
  P_Q_calculator4 : Subsystem
  P_Q_calculator5 : Subsystem
  Pmeas_1 : ToWorkspace  VariableName=PQload_1  SampleTime=-1  SaveFormat=Array
  Pmeas_2 : ToWorkspace  VariableName=PQload_2  SampleTime=-1  SaveFormat=Array
  Pmeas_3 : ToWorkspace  VariableName=PQload_3  SampleTime=-1  SaveFormat=Array
  Preq1 : Scope
  Preq2 : Scope
  Preq3 : Scope
  Scope{1..3,8..12,15..16} (10 alike) : Scope
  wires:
  [v_meas_1] -> Scope8/1
  [igen_meas_1] -> Scope1/1
  [v_meas_2] -> Scope2/1
  [igen_meas_2] -> Scope3/1
  [v_meas_1] -> P_Q_calculator/1(v)
  [igen_meas_1] -> P_Q_calculator/2(i)
  P_Q_calculator1/1(P) -> Mux1/1
  P_Q_calculator1/2(Q) -> Mux1/2
  [v_meas_2] -> P_Q_calculator1/1(v)
  [igen_meas_2] -> P_Q_calculator1/2(i)
  [v_meas_load1] -> P_Q_calculator2/1(v)
  [iload_meas_1] -> P_Q_calculator2/2(i)
  [v_meas_load2] -> P_Q_calculator3/1(v)
  [iload_meas_2] -> P_Q_calculator3/2(i)
  Mux2/1 -> Gen1 Power/1
  P_Q_calculator/1(P) -> Mux2/1
  P_Q_calculator/2(Q) -> Mux2/2
  Mux1/1 -> Gen2 Power/1
  Mux3/1 -> Load1 Power/1, Pmeas_1/1
  P_Q_calculator2/1(P) -> Mux3/1
  P_Q_calculator2/2(Q) -> Mux3/2
  Mux4/1 -> Load2 Power/1, Pmeas_2/1
  P_Q_calculator3/1(P) -> Mux4/1
  P_Q_calculator3/2(Q) -> Mux4/2
  [freq1_plot] -> Gen1_freq/1
  [freq2_plot] -> Gen2_freq/1
  [v_meas_3] -> Scope15/1
  [igen_meas_3] -> Scope16/1
  P_Q_calculator4/1(P) -> Mux5/1
  P_Q_calculator4/2(Q) -> Mux5/2
  [v_meas_3] -> P_Q_calculator4/1(v)
  [igen_meas_3] -> P_Q_calculator4/2(i)
  Mux5/1 -> Gen3 Power/1
  [freq3_plot] -> Gen3_freq/1
  [v_meas_load1] -> Scope12/1
  [iload_meas_1] -> Scope9/1
  [v_meas_load2] -> Scope10/1
  [iload_meas_2] -> Scope11/1
  [Preq1_trigger] -> Preq1/1
  [Preq2_trigger] -> Preq2/1
  [Preq3_trigger] -> Preq3/1
  [v_meas_load3] -> P_Q_calculator5/1(v)
  [iload_meas_3] -> P_Q_calculator5/2(i)
  Mux6/1 -> Load3 Power/1, Pmeas_3/1
  P_Q_calculator5/1(P) -> Mux6/1
  P_Q_calculator5/2(Q) -> Mux6/2

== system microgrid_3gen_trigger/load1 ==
  Ground1 : powerlib/Elements/Ground  DialogController=POWERSYS.PowerSysDialog  PhysicalDomain=powersysdomain  SubClassName=unknown  LeftPortType=p1  RightPortType=p1  LConnTagsString=a
  Ground2 : powerlib/Elements/Ground  DialogController=POWERSYS.PowerSysDialog  PhysicalDomain=powersysdomain  SubClassName=unknown  LeftPortType=p1  RightPortType=p1  LConnTagsString=a
  Ground3 : powerlib/Elements/Ground  DialogController=POWERSYS.PowerSysDialog  PhysicalDomain=powersysdomain  SubClassName=unknown  LeftPortType=p1  RightPortType=p1  LConnTagsString=a
  Neutral : powerlib/Elements/Neutral  DialogController=POWERSYS.PowerSysDialog  PhysicalDomain=powersysdomain  SubClassName=unknown  LeftPortType=p1  RightPortType=p1  LConnTagsString=a  NodeNumber=10
  Neutral1 : powerlib/Elements/Neutral  DialogController=POWERSYS.PowerSysDialog  PhysicalDomain=powersysdomain  SubClassName=unknown  LeftPortType=p1  RightPortType=p1  LConnTagsString=a  NodeNumber=10
  Neutral2 : powerlib/Elements/Neutral  DialogController=POWERSYS.PowerSysDialog  PhysicalDomain=powersysdomain  SubClassName=unknown  LeftPortType=p1  RightPortType=p1  LConnTagsString=a  NodeNumber=10
  a : powerlib/Elements/Series RLC Branch  DialogController=POWERSYS.PowerSysDialog  PhysicalDomain=powersysdomain  SubClassName=unknown  LeftPortType=p1  RightPortType=p1  LConnTagsString=__new0  RConnTagsString=__new0  BranchType=RL  Resistance=Rload1  Inductance=Lload1  SetiL0=off  InitialCurrent=0  Capacitance=1e-6  Setx0=off  InitialVoltage=0  Measurements=None
  b : powerlib/Elements/Series RLC Branch  DialogController=POWERSYS.PowerSysDialog  PhysicalDomain=powersysdomain  SubClassName=unknown  LeftPortType=p1  RightPortType=p1  LConnTagsString=__new0  RConnTagsString=__new0  BranchType=RL  Resistance=Rload1  Inductance=Lload1  SetiL0=off  InitialCurrent=0  Capacitance=1e-6  Setx0=off  InitialVoltage=0  Measurements=None
  c : powerlib/Elements/Series RLC Branch  DialogController=POWERSYS.PowerSysDialog  PhysicalDomain=powersysdomain  SubClassName=unknown  LeftPortType=p1  RightPortType=p1  LConnTagsString=__new0  RConnTagsString=__new0  BranchType=RL  Resistance=Rload1  Inductance=Lload1  SetiL0=off  InitialCurrent=0  Capacitance=1e-6  Setx0=off  InitialVoltage=0  Measurements=None
  a1 : PMIOPort  Port=1  Side=Left
  b1 : PMIOPort  Port=2  Side=Left
  c1 : PMIOPort  Port=3  Side=Left
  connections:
  a1/RConn1 -- a/LConn1
  b1/RConn1 -- b/LConn1
  c1/RConn1 -- c/LConn1
  Ground3/LConn1 -- c/RConn1
  Ground1/LConn1 -- b/RConn1
  Ground2/LConn1 -- a/RConn1

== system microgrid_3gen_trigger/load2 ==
  Ground1 : powerlib/Elements/Ground  DialogController=POWERSYS.PowerSysDialog  PhysicalDomain=powersysdomain  SubClassName=unknown  LeftPortType=p1  RightPortType=p1  LConnTagsString=a
  Ground2 : powerlib/Elements/Ground  DialogController=POWERSYS.PowerSysDialog  PhysicalDomain=powersysdomain  SubClassName=unknown  LeftPortType=p1  RightPortType=p1  LConnTagsString=a
  Ground3 : powerlib/Elements/Ground  DialogController=POWERSYS.PowerSysDialog  PhysicalDomain=powersysdomain  SubClassName=unknown  LeftPortType=p1  RightPortType=p1  LConnTagsString=a
  Neutral : powerlib/Elements/Neutral  DialogController=POWERSYS.PowerSysDialog  PhysicalDomain=powersysdomain  SubClassName=unknown  LeftPortType=p1  RightPortType=p1  LConnTagsString=a  NodeNumber=10
  Neutral1 : powerlib/Elements/Neutral  DialogController=POWERSYS.PowerSysDialog  PhysicalDomain=powersysdomain  SubClassName=unknown  LeftPortType=p1  RightPortType=p1  LConnTagsString=a  NodeNumber=10
  Neutral2 : powerlib/Elements/Neutral  DialogController=POWERSYS.PowerSysDialog  PhysicalDomain=powersysdomain  SubClassName=unknown  LeftPortType=p1  RightPortType=p1  LConnTagsString=a  NodeNumber=10
  a : powerlib/Elements/Series RLC Branch  DialogController=POWERSYS.PowerSysDialog  PhysicalDomain=powersysdomain  SubClassName=unknown  LeftPortType=p1  RightPortType=p1  LConnTagsString=__new0  RConnTagsString=__new0  BranchType=RL  Resistance=Rload2  Inductance=Lload2  SetiL0=off  InitialCurrent=0  Capacitance=1e-6  Setx0=off  InitialVoltage=0  Measurements=None
  b : powerlib/Elements/Series RLC Branch  DialogController=POWERSYS.PowerSysDialog  PhysicalDomain=powersysdomain  SubClassName=unknown  LeftPortType=p1  RightPortType=p1  LConnTagsString=__new0  RConnTagsString=__new0  BranchType=RL  Resistance=Rload2  Inductance=Lload2  SetiL0=off  InitialCurrent=0  Capacitance=1e-6  Setx0=off  InitialVoltage=0  Measurements=None
  c : powerlib/Elements/Series RLC Branch  DialogController=POWERSYS.PowerSysDialog  PhysicalDomain=powersysdomain  SubClassName=unknown  LeftPortType=p1  RightPortType=p1  LConnTagsString=__new0  RConnTagsString=__new0  BranchType=RL  Resistance=Rload2  Inductance=Lload2  SetiL0=off  InitialCurrent=0  Capacitance=1e-6  Setx0=off  InitialVoltage=0  Measurements=None
  a2 : PMIOPort  Port=1  Side=Left
  b2 : PMIOPort  Port=2  Side=Left
  c2 : PMIOPort  Port=3  Side=Left
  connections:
  b2/RConn1 -- b/LConn1
  c2/RConn1 -- c/LConn1
  a/LConn1 -- a2/RConn1
  Ground3/LConn1 -- c/RConn1
  Ground1/LConn1 -- b/RConn1
  Ground2/LConn1 -- a/RConn1

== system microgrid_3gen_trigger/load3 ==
  Ground1 : powerlib/Elements/Ground  DialogController=POWERSYS.PowerSysDialog  PhysicalDomain=powersysdomain  SubClassName=unknown  LeftPortType=p1  RightPortType=p1  LConnTagsString=a
  Ground2 : powerlib/Elements/Ground  DialogController=POWERSYS.PowerSysDialog  PhysicalDomain=powersysdomain  SubClassName=unknown  LeftPortType=p1  RightPortType=p1  LConnTagsString=a
  Ground3 : powerlib/Elements/Ground  DialogController=POWERSYS.PowerSysDialog  PhysicalDomain=powersysdomain  SubClassName=unknown  LeftPortType=p1  RightPortType=p1  LConnTagsString=a
  Neutral : powerlib/Elements/Neutral  DialogController=POWERSYS.PowerSysDialog  PhysicalDomain=powersysdomain  SubClassName=unknown  LeftPortType=p1  RightPortType=p1  LConnTagsString=a  NodeNumber=10
  Neutral1 : powerlib/Elements/Neutral  DialogController=POWERSYS.PowerSysDialog  PhysicalDomain=powersysdomain  SubClassName=unknown  LeftPortType=p1  RightPortType=p1  LConnTagsString=a  NodeNumber=10
  Neutral2 : powerlib/Elements/Neutral  DialogController=POWERSYS.PowerSysDialog  PhysicalDomain=powersysdomain  SubClassName=unknown  LeftPortType=p1  RightPortType=p1  LConnTagsString=a  NodeNumber=10
  a : powerlib/Elements/Series RLC Branch  DialogController=POWERSYS.PowerSysDialog  PhysicalDomain=powersysdomain  SubClassName=unknown  LeftPortType=p1  RightPortType=p1  LConnTagsString=__new0  RConnTagsString=__new0  BranchType=RL  Resistance=Rload3  Inductance=Lload3  SetiL0=off  InitialCurrent=0  Capacitance=1e-6  Setx0=off  InitialVoltage=0  Measurements=None
  b : powerlib/Elements/Series RLC Branch  DialogController=POWERSYS.PowerSysDialog  PhysicalDomain=powersysdomain  SubClassName=unknown  LeftPortType=p1  RightPortType=p1  LConnTagsString=__new0  RConnTagsString=__new0  BranchType=RL  Resistance=Rload3  Inductance=Lload3  SetiL0=off  InitialCurrent=0  Capacitance=1e-6  Setx0=off  InitialVoltage=0  Measurements=None
  c : powerlib/Elements/Series RLC Branch  DialogController=POWERSYS.PowerSysDialog  PhysicalDomain=powersysdomain  SubClassName=unknown  LeftPortType=p1  RightPortType=p1  LConnTagsString=__new0  RConnTagsString=__new0  BranchType=RL  Resistance=Rload3  Inductance=Lload3  SetiL0=off  InitialCurrent=0  Capacitance=1e-6  Setx0=off  InitialVoltage=0  Measurements=None
  a1 : PMIOPort  Port=1  Side=Left
  b1 : PMIOPort  Port=2  Side=Left
  c1 : PMIOPort  Port=3  Side=Left
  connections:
  a1/RConn1 -- a/LConn1
  b1/RConn1 -- b/LConn1
  c1/RConn1 -- c/LConn1
  Ground3/LConn1 -- c/RConn1
  Ground1/LConn1 -- b/RConn1
  Ground2/LConn1 -- a/RConn1

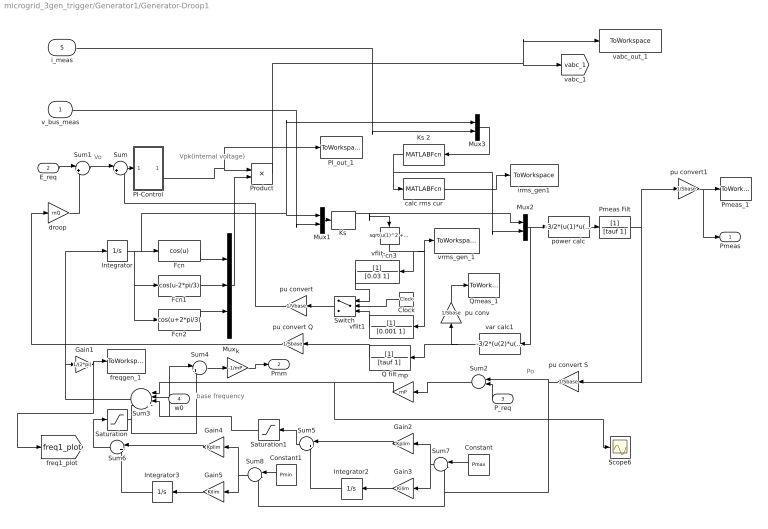
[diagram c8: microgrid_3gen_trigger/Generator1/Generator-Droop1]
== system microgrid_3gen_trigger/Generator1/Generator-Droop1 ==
  note: Vpk(internal voltage)
  note: Vo
  note: Po
  note: base frequency
  v_bus_meas : Inport
  E_req : Inport  Port=2
  P_req : Inport  Port=3
  w0 : Inport  Port=4
  i_meas : Inport  Port=5
  Clock : Clock
  Constant : Constant  Value=Pmax  OutDataType=sfix(16)  OutScaling=2^0
  Constant1 : Constant  Value=Pmin  OutDataType=sfix(16)  OutScaling=2^0
  Fcn : Fcn  Expr=cos(u)
  Fcn1 : Fcn  Expr=cos(u-2*pi/3)
  Fcn2 : Fcn  Expr=cos(u+2*pi/3)
  Fcn3 : Fcn  Expr=sqrt(u(1)^2 + u(2)^2)/sqrt(2)
  Gain1 : Gain  Gain=1/(2*pi)  ParameterDataType=sfix(16)  ParameterScaling=2^0  OutDataType=sfix(16)  OutScaling=2^0
  Gain2 : Gain  Gain=Kplim  ParameterDataType=sfix(16)  ParameterScaling=2^0  OutDataType=sfix(16)  OutScaling=2^0
  Gain3 : Gain  Gain=Kilim  ParameterDataType=sfix(16)  ParameterScaling=2^0  OutDataType=sfix(16)  OutScaling=2^0
  Gain4 : Gain  Gain=Kplim  ParameterDataType=sfix(16)  ParameterScaling=2^0  OutDataType=sfix(16)  OutScaling=2^0
  Gain5 : Gain  Gain=Kilim  ParameterDataType=sfix(16)  ParameterScaling=2^0  OutDataType=sfix(16)  OutScaling=2^0
  Integrator : Integrator
  Integrator2 : Integrator  UpperSaturationLimit=0  LowerSaturationLimit=-2*pi
  Integrator3 : Integrator  UpperSaturationLimit=2*pi  LowerSaturationLimit=0
  Ks : MATLABFcn  MATLABFcn=Ks_
  Ks 2 : MATLABFcn  MATLABFcn=Ks_
  Mux : Mux  Inputs=3
  Mux1 : Mux  Inputs=2
  Mux2 : Mux  Inputs=2
  Mux3 : Mux  Inputs=2
  PI-Control : Subsystem
  PI_out_1 : ToWorkspace  VariableName=PI_out_1  SampleTime=-1  SaveFormat=Array
  Pmeas Filt : TransferFcn  Denominator=[tauf 1]
  Pmeas_1 : ToWorkspace  VariableName=Pmeas_1  SampleTime=-1  SaveFormat=Array
  Product : Product  OutDataType=sfix(16)  OutScaling=2^0
  Q filt : TransferFcn  Denominator=[tauf 1]
  Qmeas_1 : ToWorkspace  VariableName=Qmeas_1  SampleTime=-1  SaveFormat=Array
  Saturation : Saturate  UpperLimit=2*pi  LowerLimit=0  OutDataType=fixdt(1, 16)  OutScaling=2^0
  Saturation1 : Saturate  UpperLimit=0  LowerLimit=-2*pi  OutDataType=fixdt(1, 16)  OutScaling=2^0
  Scope6 : Scope
  Sum : Sum  Inputs=|+-  OutDataType=sfix(16)  OutScaling=2^0
  Sum{1,4..6} (4 alike) : Sum  Inputs=|++  OutDataType=sfix(16)  OutScaling=2^0
  Sum2 : Sum  Inputs=|-+  OutDataType=sfix(16)  OutScaling=2^0
  Sum3 : Sum  Inputs=|++++  OutDataType=sfix(16)  OutScaling=2^0
  Sum7 : Sum  Inputs=|+-  OutDataType=sfix(16)  OutScaling=2^0
  Sum8 : Sum  Inputs=|+-  OutDataType=sfix(16)  OutScaling=2^0
  Switch : Switch  Criteria=u2 > Threshold  Threshold=2  OutDataType=fixdt(1, 16)  OutScaling=2^0
  calc rms cur : MATLABFcn  MATLABFcn=RMS_
  "droop " : Gain  Gain=mQ  ParameterDataType=sfix(16)  ParameterScaling=2^0  OutDataType=sfix(16)  OutScaling=2^0
  freqgen_1 : ToWorkspace  VariableName=freqgen_1  SampleTime=-1  SaveFormat=Array
  irms_gen1 : ToWorkspace  VariableName=irms_gen_1  SampleTime=-1  SaveFormat=Array
  k : Gain  Gain=-1/mP  ParameterDataType=sfix(16)  ParameterScaling=2^0  OutDataType=sfix(16)  OutScaling=2^0
  mp : Gain  Gain=mP  ParameterDataType=sfix(16)  ParameterScaling=2^0  OutDataType=sfix(16)  OutScaling=2^0
  power calc : Fcn  Expr=-3/2*(u(1)*u(4) + u(2)*u(5) + 2*u(3)*u(6))
  pu conv : Gain  Gain=1/Sbase  ParameterDataType=sfix(16)  ParameterScaling=2^0  OutDataType=sfix(16)  OutScaling=2^0
  pu convert : Gain  Gain=1/Vbase  ParameterDataType=sfix(16)  ParameterScaling=2^0  OutDataType=sfix(16)  OutScaling=2^0
  pu convert Q : Gain  Gain=1/Sbase  ParameterDataType=sfix(16)  ParameterScaling=2^0  OutDataType=sfix(16)  OutScaling=2^0
  pu convert S : Gain  Gain=1/Sbase  ParameterDataType=sfix(16)  ParameterScaling=2^0  OutDataType=sfix(16)  OutScaling=2^0
  pu convert1 : Gain  Gain=1/Sbase  ParameterDataType=sfix(16)  ParameterScaling=2^0  OutDataType=sfix(16)  OutScaling=2^0
  vabc_out_1 : ToWorkspace  VariableName=vabc_out_1  SampleTime=-1  SaveFormat=Array
  var calc1 : Fcn  Expr=-3/2*(u(2)*u(4) - u(1)*u(5))
  vflit : TransferFcn  Denominator=[0.03 1]
  vflit1 : TransferFcn  Denominator=[0.001 1]
  vrms_gen_1 : ToWorkspace  VariableName=vrms_gen_1  SampleTime=-1  SaveFormat=Array
  Pmeas : Outport  OutDataType=fixdt(1, 16)  OutScaling=2^0
  Pmm : Outport  Port=2  OutDataType=fixdt(1, 16)  OutScaling=2^0
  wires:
  Integrator/1 -> Fcn1/1, Fcn2/1, Fcn/1, Mux1/1, Mux3/1
  Fcn/1 -> Mux/1
  Fcn1/1 -> Mux/2
  Fcn2/1 -> Mux/3
  Mux/1 -> Product/2
  Sum1/1 -> Sum/1
  pu convert/1 -> Sum/2
  "droop "/1 -> Sum1/2
  pu convert S/1 -> Sum2/1, Sum7/2, Sum8/2
  Sum2/1 -> mp/1
  mp/1 -> Sum3/1, Scope6/1
  Sum3/1 -> Integrator/1, Gain1/1
  pu convert Q/1 -> "droop "/1
  Q filt/1 -> pu convert Q/1
  E_req/1 -> Sum1/1
  P_req/1 -> Sum2/2
  w0/1 -> Sum3/2
  PI-Control/1(Out1) -> Product/1, PI_out_1/1
  Gain3/1 -> Integrator2/1
  Integrator2/1 -> Sum5/2
  Gain2/1 -> Sum5/1
  Gain5/1 -> Integrator3/1
  Integrator3/1 -> Sum6/2
  Gain4/1 -> Sum6/1
  Sum7/1 -> Gain2/1, Gain3/1
  Sum8/1 -> Gain5/1, Gain4/1
  Constant/1 -> Sum7/1
  Constant1/1 -> Sum8/1
  Sum/1 -> PI-Control/1(In1)
  calc rms cur/1 -> irms_gen1/1
  Mux3/1 -> Ks 2/1
  var calc1/1 -> Q filt/1, pu conv/1
  Ks 2/1 -> Mux2/2, calc rms cur/1
  Mux2/1 -> power calc/1, var calc1/1
  Mux1/1 -> Ks/1
  Fcn3/1 -> vflit/1, vflit1/1, vrms_gen_1/1
  Gain1/1 -> freqgen_1/1, [freq1_plot]
  Ks/1 -> Mux2/1, Fcn3/1
  v_bus_meas/1 -> Mux1/2
  pu convert1/1 -> Pmeas/1, Pmeas_1/1
  pu conv/1 -> Qmeas_1/1
  i_meas/1 -> Mux3/2
  Product/1 -> [vabc_1], vabc_out_1/1
  Sum6/1 -> Saturation/1
  Saturation/1 -> Sum3/4, Sum4/2
  Sum5/1 -> Saturation1/1
  Saturation1/1 -> Sum3/3, Sum4/1
  Sum4/1 -> k/1
  k/1 -> Pmm/1
  power calc/1 -> Pmeas Filt/1
  Pmeas Filt/1 -> pu convert S/1, pu convert1/1
  vflit/1 -> Switch/1
  Switch/1 -> pu convert/1
  vflit1/1 -> Switch/3
  Clock/1 -> Switch/2

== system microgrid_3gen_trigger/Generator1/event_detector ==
  phi : Inport
  z : Inport  Port=2
  Demux : Demux  Outputs=2
  Mux2 : Mux  Inputs=2
  S-Function : S-Function  FunctionName=trigger_block  EnableBusSupport=off
  phi_hat : Outport
  tsamp : Outport  Port=2
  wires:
  Mux2/1 -> S-Function/1
  z/1 -> Mux2/2
  phi/1 -> Mux2/1
  Demux/2 -> tsamp/1
  Demux/1 -> phi_hat/1
  S-Function/1 -> Demux/1

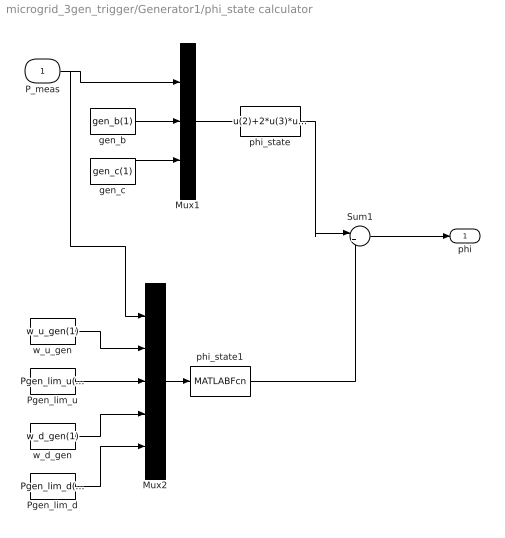
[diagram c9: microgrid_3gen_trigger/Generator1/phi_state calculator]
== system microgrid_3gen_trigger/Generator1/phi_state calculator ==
  P_meas : Inport
  Mux1 : Mux  Inputs=3
  Mux2 : Mux  Inputs=5
  Pgen_lim_d : Constant  Value=Pgen_lim_d(1)  OutDataType=sfix(16)  OutScaling=2^0
  Pgen_lim_u : Constant  Value=Pgen_lim_u(1)  OutDataType=sfix(16)  OutScaling=2^0
  Sum1 : Sum  Inputs=|++  OutDataType=sfix(16)  OutScaling=2^0
  gen_b : Constant  Value=gen_b(1)  OutDataType=sfix(16)  OutScaling=2^0
  gen_c : Constant  Value=gen_c(1)  OutDataType=sfix(16)  OutScaling=2^0
  phi_state : Fcn  Expr=u(2)+2*u(3)*u(1)
  phi_state1 : MATLABFcn  MATLABFcn=phi_state
  w_d_gen : Constant  Value=w_d_gen(1)  OutDataType=sfix(16)  OutScaling=2^0
  w_u_gen : Constant  Value=w_u_gen(1)  OutDataType=sfix(16)  OutScaling=2^0
  phi : Outport  OutDataType=fixdt(1, 16)  OutScaling=2^0
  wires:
  Mux1/1 -> phi_state/1
  gen_c/1 -> Mux1/3
  P_meas/1 -> Mux1/1, Mux2/1
  gen_b/1 -> Mux1/2
  Mux2/1 -> phi_state1/1
  w_u_gen/1 -> Mux2/2
  Pgen_lim_u/1 -> Mux2/3
  w_d_gen/1 -> Mux2/4
  Pgen_lim_d/1 -> Mux2/5
  phi_state1/1 -> Sum1/2
  phi_state/1 -> Sum1/1
  Sum1/1 -> phi/1
